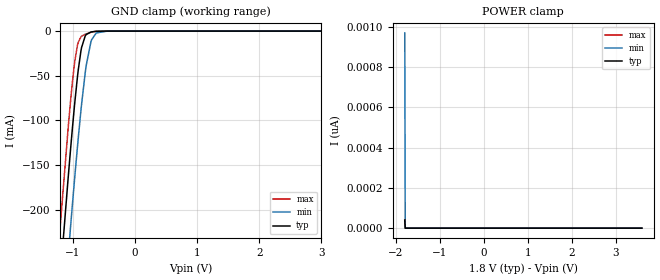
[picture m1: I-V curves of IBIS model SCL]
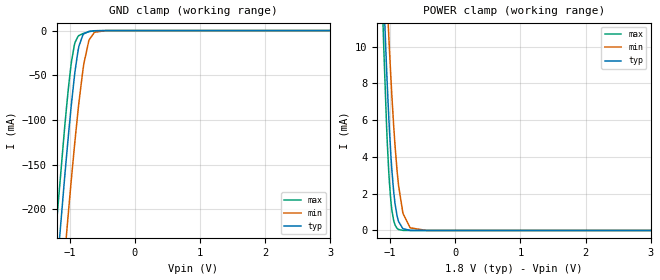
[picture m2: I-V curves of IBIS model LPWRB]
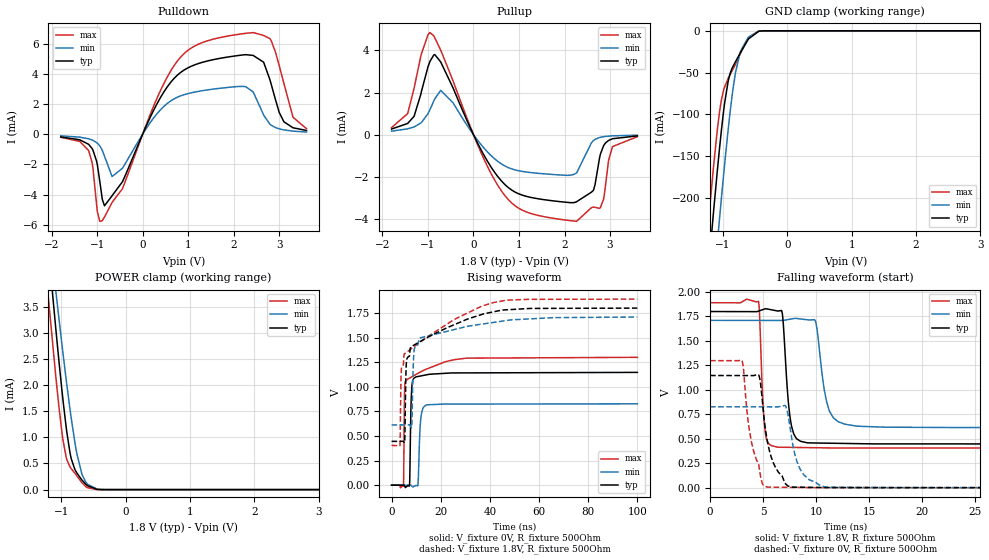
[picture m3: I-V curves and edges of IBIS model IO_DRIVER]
| Texas Instruments Incorporated
| Marketing part#   Voltage Range   Package-type   #pins/pkg drawing
| LDC2114YFD   1.71V - 1.89V   DSBGA   16-pin YFD
[IBIS Ver]   4.1
[File name]   ldc2114.ibs
[File Rev]   1.0
[Date]   05/20/2016
[Source]   Model built from spectre simulations at:
   Texas Instruments Incorporated.
   Analog-eLab, HPA
   12500 TI Blvd
   Dallas, TX -75243
   For Support e-mail: elab_ibis@list.ti.com
[Notes]   Revision History
   Rev 1.0: 05/20/2016
   -Pullup and Pulldown non-monotonic for IO_DRIVER
   -Pulldown non-monotonic for SDA
   - ccomp values are based on PVT settings:
   MIN: Low Voltage, High Temperature, Weak Process
   TYP: Nominal Voltage, Nominal Temperature, Nominal Process
   MAX: High Voltage, Low Temperature, Fast Process
   - C_comp although listed in numerical order of value are obtained from varying PVT conditions.
   For PVT conditions for each specific value, refer to the buffer description under respective [Model].
   IBIS model user is responsible for using appropriate C_comp to simulate for Signal Integrity.
[Disclaimer]  This model is designed as an aid for customers of Texas Instruments
 TI and its licensors and suppliers make no warranties, either expressed
 or implied, with respect to this  model, including the warranties of
 merchantability or fitness for a particular purpose.
 The model is provided solely on an "as is" basis. The entire risk as to
 its quality and performance is with the customer.
[Copyright] (C)Copyright 2016 Texas Instruments Incorporated.
   All rights reserved.
[Component]   LDC2114YFD
[Manufacturer]  Texas Instruments Incorporated
[Package]   |16-pin YFD DSBGA package
|   typ   min   max
R_pkg   0.005   0.005   0.005
L_pkg   0.20nH   0.2nH   0.2nH
C_pkg   0.6pF   0.6pF   0.6pF
[Pin]   signal_name   model_name   R_pin   L_pin   C_pin
A1   IN3   NC   0.005   0.2nH   0.6pF
A2   IN2   NC   0.005   0.2nH   0.6pF
A3   IN1   NC   0.005   0.2nH   0.6pF
A4   GND   GND   0.005   0.2nH   0.6pF
B1   IN4   NC   0.005   0.2nH   0.6pF
B2   INTB   IO_DRIVER   0.005   0.2nH   0.6pF
B3   OUT4   IO_DRIVER   0.005   0.2nH   0.6pF
B4   OUT3   IO_DRIVER   0.005   0.2nH   0.6pF
C1   VCC   POWER   0.005   0.2nH   0.6pF
C2   LPWRB   LPWRB   0.005   0.2nH   0.6pF
C3   SDA   SDA   0.005   0.2nH   0.6pF
C4   OUT2   IO_DRIVER   0.005   0.2nH   0.6pF
D1   GND   GND   0.005   0.2nH   0.6pF
D2   COM   NC   0.005   0.2nH   0.6pF
D3   SCL   SCL   0.005   0.2nH   0.6pF
D4   OUT1   IO_DRIVER   0.005   0.2nH   0.6pF
| Models and submodels in the file (4): SCL (Input), LPWRB (Input), IO_DRIVER (3-state), SDA (I/O_open_drain)
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|   Model SCL
[Model]   SCL
Model_type   Input
Vinl = .513
Vinh = 1.323
|   typ   min   max
|   (nom PVT)   (slow PVT)   (fast PVT)
C_comp   0.816p   0.784p   0.852p
[Voltage Range]   1.8   1.71   1.89
[Temperature Range]   27   125   -40
[Power Clamp Reference]   1.8   1.71   1.89
[GND Clamp Reference]   0   0   0
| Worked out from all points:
|   GND clamp passes 1 mA (typ) near -0.71 V on its own axis
[GND Clamp]
|   Voltage   I(typ)   I(min)   I(max)
-1.8V     -838.3mA   -923.5mA   -783.9mA
-1.206V   -278.1mA   -367mA     -220.8mA
-1.19V    -263.6mA   -352.4mA   -206.2mA
-1.076V   -164.7mA   -252.6mA   -108.9mA
-1.039V   -133.5mA   -220.3mA   -79.36mA
-968.4mV  -79.49mA   -162.5mA   -33.35mA
-919.8mV  -47.32mA   -124.7mA   -14.14mA
-860.4mV  -18.58mA   -82.34mA   -5.802mA
-784.8mV  -3.863mA   -38.34mA   -3.123mA
-709.2mV  -1.067mA   -11.92mA   -1.361mA
-622.8mV  -216uA     -2.053mA   -227.9uA
3.6V      0A         0A         0A
[POWER Clamp]
|   Voltage   I(typ)   I(min)   I(max)
-1.8V     40.1pA     968.4pA    39.81pA
-1.789V   0A         0A         0A
-1.784V   0A         0A         0A
3.6V      0A         0A         0A
|   Model LPWRB
[Model]   LPWRB
Model_type   Input
Vinl = .513
Vinh = 1.323
|   typ   min   max
|   (nom PVT)   (slow PVT)   (fast PVT)
C_comp   1.179p   1.170p   1.187p
[Voltage Range]   1.8   1.71   1.89
[Temperature Range]   27   125   -40
[Power Clamp Reference]   1.8   1.71   1.89
[GND Clamp Reference]   0   0   0
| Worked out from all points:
|   GND clamp passes 1 mA (typ) near -0.70 V on its own axis
|   POWER clamp passes 1 mA (typ) near -0.90 V on its own axis
[GND Clamp]
|   Voltage   I(typ)   I(min)   I(max)
-1.8V     -838.6mA   -924mA     -784.2mA
-1.206V   -278.7mA   -367.7mA   -221.2mA
-1.19V    -264.2mA   -353.1mA   -206.7mA
-1.076V   -165.4mA   -253.4mA   -109.5mA
-1.039V   -134.2mA   -221.2mA   -79.93mA
-973.8mV  -84.15mA   -167.8mA   -36.79mA
-925.2mV  -51.35mA   -129.8mA   -15.91mA
-855mV    -17.26mA   -79.83mA   -5.508mA
-779.4mV  -3.586mA   -36.74mA   -2.997mA
-703.8mV  -984.8uA   -11.29mA   -1.252mA
-617.4mV  -192.8uA   -1.924mA   -197.5uA
3.6V      0A         0A         0A
[POWER Clamp]
|   Voltage   I(typ)   I(min)   I(max)
-1.8V     98.48mA    89.24mA    116.8mA
-1.109V   13.69mA    17.65mA    11.12mA
-1.098V   12.65mA    16.71mA    9.903mA
-1.055V   8.756mA    13.13mA    5.634mA
-1.022V   6.231mA    10.64mA    3.235mA
-1.012V   5.481mA    9.855mA    2.614mA
-946.8mV  2.13mA     5.72mA     549.6uA
-871.2mV  489.6uA    2.445mA    54.56uA
-801mV    93.73uA    908.1uA    5.457uA
-693mV    5.767uA    145.7uA    331.5nA
-444.6mV  17.3nA     1.139uA    57.09nA
3.6V      0A         0A         0A
|   Model IO_DRIVER
[Model]   IO_DRIVER
Model_type   3-state
Polarity   Non-Inverting
Vmeas = 0.9
Vref = 1.8
Cref = 15pF
Rref = 500
|   typ   min   max
|   (nom PVT)   (slow PVT)   (fast PVT)
C_comp   1.123p   1.113p   1.127p
|C_comp (High state)   1.149p   1.132p   1.167p
|C_comp (Low state)   1.123p   1.113p   1.127p
[Voltage Range]   1.8   1.71   1.89
[Temperature Range]   27   125   -40
[Pullup Reference]   1.8   1.71   1.89
[Pulldown Reference]   0   0   0
[Power Clamp Reference]   1.8   1.71   1.89
[GND Clamp Reference]   0   0   0
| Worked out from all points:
|   slope of the pulldown table from 0 to 0.27 V, typ, clamps not added: 154 ohm
|   slope of the pullup table from 0 to 0.27 V, typ, clamps not added: 241 ohm
|   GND clamp passes 1 mA (typ) near -0.45 V on its own axis
|   POWER clamp passes 1 mA (typ) near -0.90 V on its own axis
|   falling waveform, V_fixture 1.8V, R_fixture 500Ohm: 20-80 % time 558ps typ, 891ps min, 355ps max; typ from 1.8 V to 0.446 V
|   rising waveform, V_fixture 0V, R_fixture 500Ohm: 20-80 % time 564ps typ, 828ps min, 457ps max; typ from 0 V to 1.15 V
|   rising waveform, V_fixture 1.8V, R_fixture 500Ohm: 20-80 % time 11.2ns typ, 2.99ns min, 16.3ns max; typ from 0.445 V to 1.8 V
|   falling waveform, V_fixture 0V, R_fixture 500Ohm: 20-80 % time 1.17ns typ, 1.17ns min, 1.21ns max; typ from 1.15 V to 0 V
[Pulldown]
|   Voltage   I(typ)   I(min)   I(max)
-1.8V     -182.9uA   -109.8uA   -208.1uA
-1.19V    -668.3uA   -305.1uA   -1.075mA
-1.093V   -1.054mA   -408.8uA   -2.24mA
-995.4mV  -2.034mA   -597.5uA   -5.131mA
-887.4mV  -4.309mA   -1.065mA   -5.732mA
-671.4mV  -4.075mA   -2.806mA   -4.515mA
781.2mV   3.956mA    2.471mA    4.911mA
2.428V    5.214mA    2.799mA    6.728mA
2.822V    3.324mA    599.2uA    6.207mA
3.001V    1.434mA    350.7uA    4.535mA
3.303V    422.6uA    200.7uA    1.118mA
3.6V      244.1uA    140.3uA    362.8uA
[GND Clamp]
|   Voltage   I(typ)   I(min)   I(max)
-1.8V     -827.3mA   -916.8mA   -771.2mA
-1.238V   -297.5mA   -387.9mA   -240.6mA
-1.195V   -259.1mA   -348.9mA   -203mA
-1.147V   -216.8mA   -305.6mA   -162.6mA
-1.055V   -141.8mA   -226mA     -97.9mA
-995.4mV  -99.55mA   -176.8mA   -72.71mA
-919.8mV  -60.6mA    -118.8mA   -57.06mA
-806.4mV  -37.16mA   -50.36mA   -40.22mA
-725.4mV  -25.72mA   -24.1mA    -26.48mA
-612mV    -10.73mA   -8.452mA   -9.031mA
-444.6mV  -579.4uA   -559.9uA   -199.6uA
3.6V      0A         0A         0A
[Pullup]
|   Voltage   I(typ)   I(min)   I(max)
-1.8V     267.7uA    168.2uA    335.7uA
-1.449V   531.1uA    274.8uA    996.4uA
-1.309V   863.8uA    365.6uA    2.166mA
-957.6mV  3.475mA    1.182mA    4.851mA
-720mV    3.454mA    2.106mA    4.012mA
365.4mV   -1.467mA   -949.1uA   -1.759mA
1.067V    -2.869mA   -1.743mA   -3.581mA
2.255V    -3.196mA   -1.832mA   -4.114mA
2.633V    -2.646mA   -284.2uA   -3.439mA
2.768V    -1.122mA   -135.7uA   -3.503mA
3.055V    -192.2uA   -55.55uA   -566uA
3.6V      -57.86uA   -23.38uA   -95.67uA
[POWER Clamp]
|   Voltage   I(typ)   I(min)   I(max)
-1.8V     13.18mA    12.18mA    12.27mA
-1.206V   4.681mA    5.154mA    3.739mA
-1.184V   4.387mA    4.908mA    3.447mA
-1.082V   3.025mA    3.76mA     2.114mA
-973.8mV  1.709mA    2.603mA    946.8uA
-919.8mV  1.146mA    2.056mA    597.5uA
-860.4mV  675.2uA    1.492mA    426uA
-757.8mV  315.9uA    683.1uA    261uA
-682.2mV  186.7uA    305.2uA    136.6uA
-590.4mV  72.85uA    100.3uA    34.8uA
-336.6mV  227.8nA    1.21uA     12.52nA
3.6V      0A         0A         0A
[Ramp]
R_load = 500
|   typ   min   max
dV/dt_r   0.68749/5.57061e-10   0.495866/8.18342e-10   0.779287/4.51074e-10
dV/dt_f   0.812325/5.56824e-10   0.65809/8.75908e-10   0.891352/3.55302e-10
[Falling Waveform]
V_fixture = 1.8V
V_fixture_min = 1.71V
V_fixture_max = 1.89V
R_fixture = 500Ohm
C_fixture = 0F
|   Time   V(typ)   V(min)   V(max)
0s        1.8V       1.71V      1.89V
4.563ns   1.804V     1.709V     1.904V
5.21ns    1.828V     1.709V     563.2mV
6.326ns   1.807V     1.709V     416.3mV
6.821ns   1.773V     1.709V     414.4mV
7.699ns   622.6mV    1.725V     413.1mV
9.152ns   460.2mV    1.716V     410.9mV
11.29ns   455.7mV    775.9mV    407.6mV
13.73ns   451.7mV    631.8mV    407.1mV
100ns     446.1mV    613.2mV    404.4mV
[Rising Waveform]
V_fixture = 0V
V_fixture_min = 0V
V_fixture_max = 0V
R_fixture = 500Ohm
C_fixture = 0F
|   Time   V(typ)   V(min)   V(max)
0s        1.102nV    38.54nV    75.36nV
4.837ns   459.5uV    283.9uV    -11.79mV
5.389ns   -11.6mV    316.3uV    1.019V
7.27ns    -9.337mV   426.7uV    1.087V
7.889ns   773.6mV    463uV      1.096V
8.274ns   1.002V     -8.273mV   1.101V
10.68ns   1.104V     -4.323mV   1.135V
11.56ns   1.108V     562.5mV    1.148V
14.39ns   1.122V     816.6mV    1.181V
100ns     1.146V     826.4mV    1.299V
[Rising Waveform]
V_fixture = 1.8V
V_fixture_min = 1.71V
V_fixture_max = 1.89V
R_fixture = 500Ohm
C_fixture = 0F
|   Time   V(typ)   V(min)   V(max)
0s        445.1mV    611.7mV    404.4mV
3.407ns   445.8mV    612.4mV    400.3mV
3.943ns   445.9mV    612.5mV    1.159V
5.169ns   433.2mV    612.8mV    1.332V
5.997ns   1.234V     612.9mV    1.348V
7.817ns   1.404V     596.1mV    1.382V
8.237ns   1.41V      608.7mV    1.39V
9.511ns   1.428V     1.405V     1.413V
24.44ns   1.619V     1.574V     1.666V
100ns     1.799V     1.708V     1.89V
[Falling Waveform]
|Gnd
V_fixture = 0V
V_fixture_min = 0V
V_fixture_max = 0V
R_fixture = 500Ohm
C_fixture = 0F
|   Time   V(typ)   V(min)   V(max)
0s        1.147V     827.6mV    1.299V
3.014ns   1.146V     827.3mV    1.297V
3.704ns   1.146V     827.2mV    590.2mV
4.599ns   1.149V     827.1mV    229.5mV
4.913ns   907.3mV    827mV      48.91mV
5.412ns   472.1mV    827mV      7.683mV
7.358ns   18.01mV    740.3mV    5.211mV
8.507ns   6.362mV    188.3mV    3.922mV
10.98ns   2.988mV    7.069mV    2.624mV
100ns     9.313uV    61.37uV    75.36nV
